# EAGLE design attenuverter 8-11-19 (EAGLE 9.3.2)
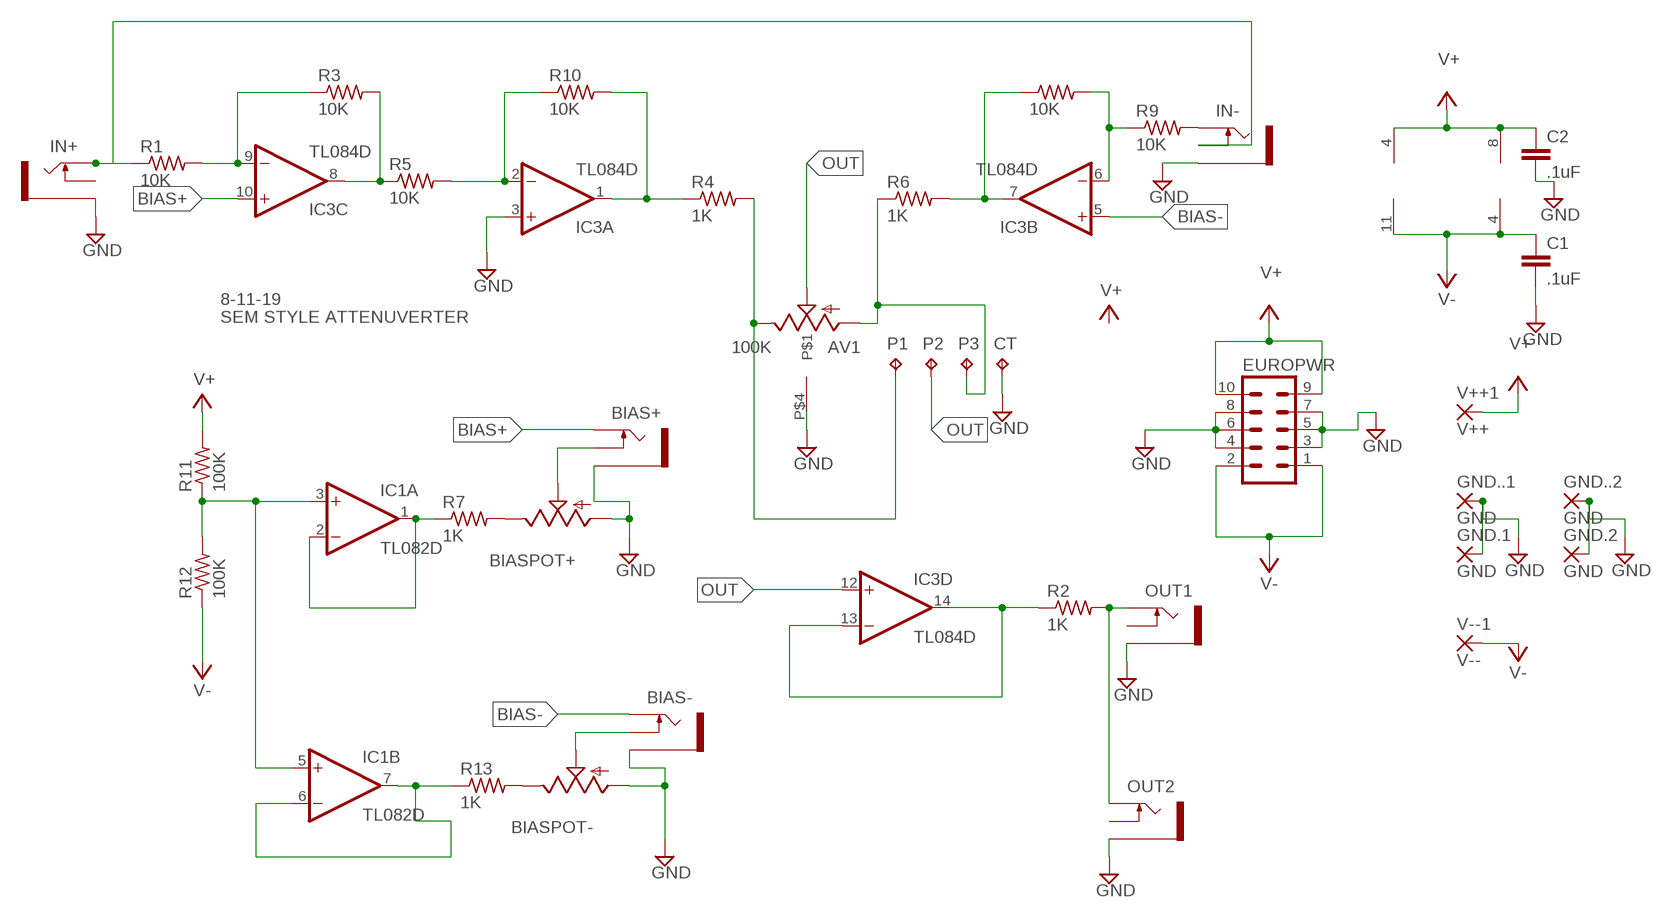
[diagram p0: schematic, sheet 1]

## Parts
AV1  100K  ALPSRK11K114  [ALPSCENTERTAP]
BIAS+  THONKICONNOLD  [THONKICONN]
BIAS-  THONKICONNOLD  [THONKICONN]
BIASPOT+  9MM_SNAP-IN_POT_  [9MM_SNAP-IN_POT]
BIASPOT-  9MM_SNAP-IN_POT_  [9MM_SNAP-IN_POT]
C1  .1uF  C5/3.5  [C5B3.5]
C2  .1uF  C5/3.5  [C5B3.5]
CT  TPPAD1-13  [P1-13]
EUROPWR  EURO_POWER_HEADERREGULAR  [EURO_POWER_HEADER]
GND.1  GND  1,6/0,8  [1,6/0,8]
GND.2  GND  1,6/0,8  [1,6/0,8]
GND..1  GND  1,6/0,8  [1,6/0,8]
GND..2  GND  1,6/0,8  [1,6/0,8]
IC1  TL082D  [SO08]
IC3  TL084D  [SO14]
IN+  THONKICONNOLD  [THONKICONN]
IN-  THONKICONNOLD  [THONKICONN]
OUT1  THONKICONNOLD  [THONKICONN]
OUT2  THONKICONNOLD  [THONKICONN]
P1  TPPAD1-13  [P1-13]
P2  TPPAD1-13  [P1-13]
P3  TPPAD1-13  [P1-13]
R1  10K  R-US_0204/7  [0204/7]
R2  1K  R-US_0204/7  [0204/7]
R3  10K  R-US_0204/7  [0204/7]
R4  1K  R-US_0204/7  [0204/7]
R5  10K  R-US_0204/7  [0204/7]
R6  1K  R-US_0204/7  [0204/7]
R7  1K  R-US_0204/7  [0204/7]
R8  10K  R-US_0204/7  [0204/7]
R9  10K  R-US_0204/7  [0204/7]
R10  10K  R-US_0204/7  [0204/7]
R11  100K  R-US_0204/7  [0204/7]
R12  100K  R-US_0204/7  [0204/7]
R13  1K  R-US_0204/7  [0204/7]
V++1  V++  1,6/0,8  [1,6/0,8]
V--1  V--  1,6/0,8  [1,6/0,8]

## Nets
BIAS+: BIAS+.P$3_TIP(TIP) IC3.10(C:+IN)
BIAS-: BIAS-.P$3_TIP(TIP) IC3.5(B:+IN)
GND: AV1.P$4 BIAS+.P$1_SLEEVE(SLEEVE) BIAS-.P$1_SLEEVE(SLEEVE) BIASPOT+.1(A) BIASPOT-.1(A) C1.2 C2.2 CT.TP EUROPWR.3 EUROPWR.4 EUROPWR.5 EUROPWR.6 EUROPWR.7 EUROPWR.8 GND.1.1(P) GND.2.1(P) GND..1.1(P) GND..2.1(P) IC3.3(A:+IN) IN+.P$1_SLEEVE(SLEEVE) IN-.P$1_SLEEVE(SLEEVE) OUT1.P$1_SLEEVE(SLEEVE) OUT2.P$1_SLEEVE(SLEEVE)
N$1: IC3.6(B:-IN) R8.2 R9.1
N$2: IC1.3(A:+IN) IC1.5(B:+IN) R11.1 R12.2
N$3: IC3.7(B:OUT) R6.2 R8.1
N$4: IC1.1(A:OUT) IC1.2(A:-IN) R7.1
N$5: AV1.P$1(HIGH) P1.TP R4.2
N$6: IC1.6(B:-IN) IC1.7(B:OUT) R13.1
N$7: BIASPOT-.3(E) R13.2
N$8: IN-.P$3_TIP(TIP) R9.2
N$9: BIAS+.P$2_SWITCH(SWITCH) BIASPOT+.2(S)
N$10: BIAS-.P$2_SWITCH(SWITCH) BIASPOT-.2(S)
N$11: IC3.9(C:-IN) R1.2 R3.1
N$12: IC3.13(D:-IN) IC3.14(D:OUT) R2.1
N$13: AV1.P$3(LOW) P3.TP R6.1
N$14: BIASPOT+.3(E) R7.2
N$16: IC3.8(C:OUT) R3.2 R5.1
N$17: IC3.2(A:-IN) R5.2 R10.1
N$18: IC3.1(A:OUT) R4.1 R10.2
N$19: IN+.P$3_TIP(TIP) IN-.P$2_SWITCH(SWITCH) R1.1
N$20: OUT1.P$3_TIP(TIP) OUT2.P$3_TIP(TIP) R2.2
OUT: AV1.P$2(WIPER) IC3.12(D:+IN) P2.TP
V+: C2.1 EUROPWR.9 EUROPWR.10 IC1.8(P:V+) IC3.4(P:V+) R11.2 V++1.1(P)
V-: C1.1 EUROPWR.1 EUROPWR.2 IC1.4(P:V-) IC3.11(P:V-) R12.1 V--1.1(P)
Unconnected: IN+.P$2_SWITCH(SWITCH) OUT1.P$2_SWITCH(SWITCH) OUT2.P$2_SWITCH(SWITCH)

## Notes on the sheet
- 8-11-19
- SEM STYLE ATTENUVERTER

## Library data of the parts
AV1 = MusicThingModular-CL:ALPSRK11K114: ALPS Pot with center tap ground
BIAS+ BIAS- IN+ IN- OUT1 OUT2 = MusicThingModular:THONKICONN: 3.5mm socket for Eurorack modular synths
BIASPOT+ BIASPOT- = MusicThingModular:9MM_SNAP-IN_POT: 9mm vertical snap-in pot, Alpha / Panasonic style
C1 C2 = capacitor-wima:C: CAPACITOR
CT P1-P3 = testpad-CL:TP: Test pad NO NAME
EUROPWR = MusicThingModular:EURO_POWER_HEADER: Power Header 10 pin power header for Eurorack Power Supplies Variants with fatter pads for easier soldering, and the LOCK variant which has 5mil offset pins to hold the component in place before soldering
GND.1 GND.2 GND..1 GND..2 V++1 V--1 = wirepad-NONAMES:1,6/0,8: THROUGH-HOLE PAD
IC1 = linear:TL082: OP AMP Data sheet; DATA_SHEET: <a href="http://www.ti.com/lit/ds/symlink/tl084a.pdf"> Data sheet </a>
IC3 = linear:TL084: OP AMP
R1-R13 = rcl:R-US_: RESISTOR, American symbol

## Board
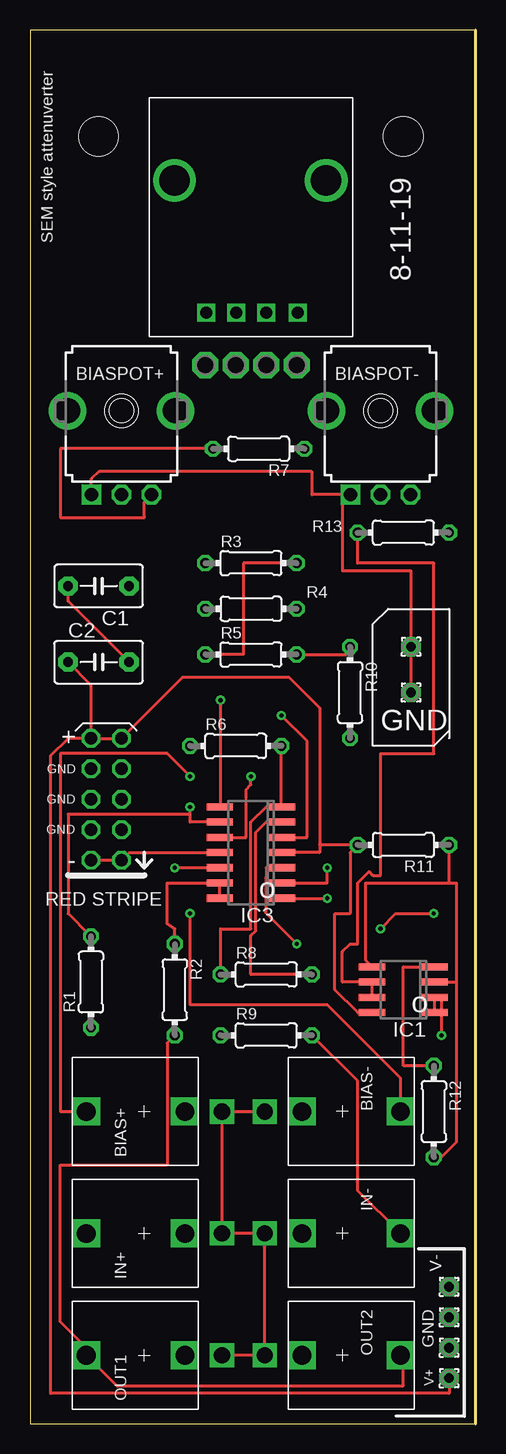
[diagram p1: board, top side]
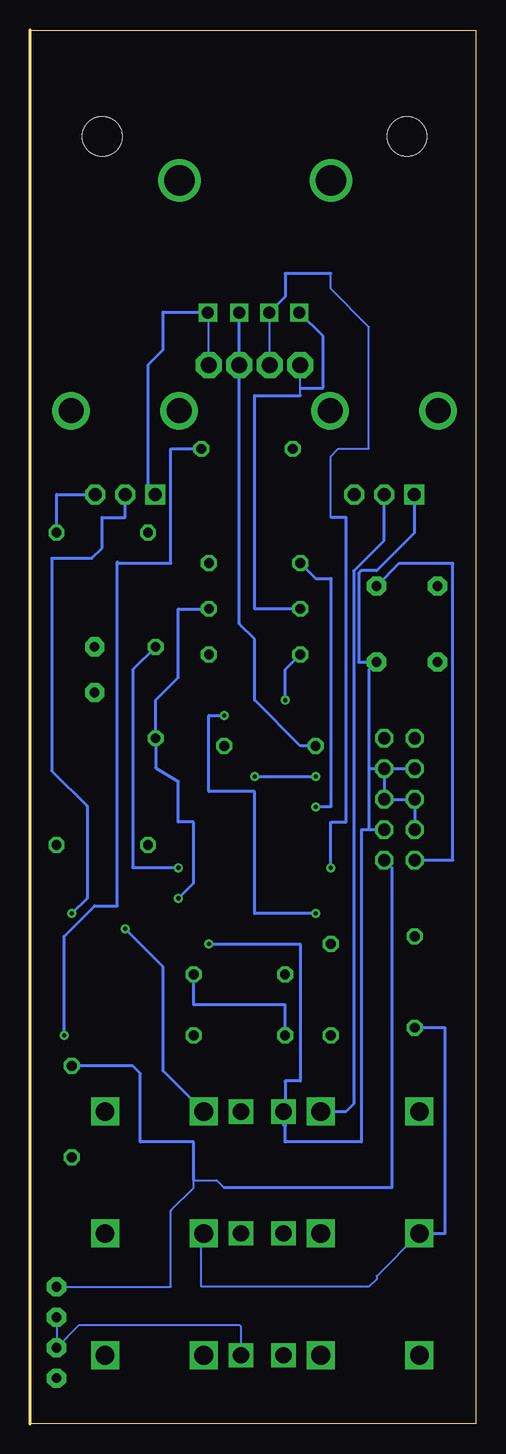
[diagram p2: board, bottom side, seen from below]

Size 37.14 x 116.19 mm. Coordinates in mm from the lower left corner, seen from the top.
Outline: 0,0 37.14,0 37.14,116.19 0,116.19 0,0
Copper layers (1*16): Top 0.035mm / dielectric 1.5mm / Bottom 0.035mm
Design rules "default": minimum track width 6mil, minimum drill 0.35mm, track to track 6mil, track to pad 6mil, pad to pad 6mil, via to via 6mil, smd to smd 6mil, copper to edge 40mil, drill to drill 6mil, minimum pad ring 10mil, minimum via ring 8mil, stop-mask expansion 4mil, vias tented up to drill 0mil, thermal gap 10mil
Holes 3.3 mm at 5.71,107.31 31.11,107.31

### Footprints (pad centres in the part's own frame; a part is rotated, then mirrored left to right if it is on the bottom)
ALPSCENTERTAP = drill 1 square: P$1 10.238,3.746; P$2 12.738,3.746; P$3 15.238,3.746; P$4 17.857,3.746 | drill 2.54: P$5 7.603,14.746; P$6 20.238,14.746
THONKICONN = drill 1.35 square: P$1_SLEEVE 0,-6.48 | drill 1.55 square: P$2_SWITCH 0,-3.38; P$3_TIP 0,4.84
9MM_SNAP-IN_POT = drill 1.1 square: 1 -2.5,-7 | drill 1.1 octagon: 2 0,-7; 3 2.5,-7 | drill 2.1 pad 2.794: CHASSIS1 -4.5,0; CHASSIS2 4.5,0
C5B3.5 = drill 0.813 pad 1.6 octagon: 1 -2.54,0; 2 2.54,0
P1-13 = drill 1.321 pad 2.159 octagon: TP 0,0
EURO_POWER_HEADER = drill 1.016 octagon: 1 -5.08,-1.27; 2 -5.08,1.27; 3 -2.54,-1.27; 4 -2.54,1.27; 5 0,-1.27; 6 0,1.27; 7 2.54,-1.27; 8 2.54,1.27; 9 5.08,-1.27; 10 5.08,1.27
1,6/0,8 = drill 0.813 pad 1.6 octagon: 1 0,0
SO08 = smd 0.6 x 2.2: 1 -1.905,-2.6; 2 -0.635,-2.6; 3 0.635,-2.6; 4 1.905,-2.6; 5 1.905,2.6; 6 0.635,2.6; 7 -0.635,2.6; 8 -1.905,2.6
SO14 = smd 0.6 x 2.2: 1 -3.81,-2.6; 2 -2.54,-2.6; 3 -1.27,-2.6; 4 0,-2.6; 5 1.27,-2.6; 6 2.54,-2.6; 7 3.81,-2.6; 8 3.81,2.6; 9 2.54,2.6; 10 1.27,2.6; 11 0,2.6; 12 -1.27,2.6; 13 -2.54,2.6; 14 -3.81,2.6
0204/7 = drill 0.813 octagon: 1 -3.81,0; 2 3.81,0

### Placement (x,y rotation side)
AV1  4.45,88.9 0 top
BIAS+  9.53,26.04 90 top
BIAS-  26.04,26.04 270 top
BIASPOT+  7.62,84.45 0 top
BIASPOT-  29.21,84.45 0 top
C1  5.71,69.85 180 top
C2  5.71,63.5 0 top
CT  22.23,88.27 0 top
EUROPWR  6.35,52.07 90 top
GND.1  34.92,8.89 90 top
GND.2  31.75,64.77 0 top
GND..1  34.92,6.35 90 top
GND..2  31.75,60.96 0 top
IC1  31.11,36.19 90 top
IC3  18.41,47.62 90 top
IN+  9.53,15.88 90 top
IN-  26.04,15.88 270 top
OUT1  9.53,5.71 90 top
OUT2  26.04,5.71 270 top
P1  14.61,88.27 0 top
P2  17.14,88.27 0 top
P3  19.68,88.27 0 top
R1  5.08,36.83 90 top
R2  12.07,36.19 270 top
R3  18.41,71.75 0 top
R4  18.41,67.94 180 top
R5  18.41,64.13 0 top
R6  17.14,56.52 0 top
R7  19.05,81.28 180 top
R8  19.68,37.47 0 top
R9  19.68,32.39 0 top
R10  26.67,60.96 270 top
R11  31.11,48.26 180 top
R12  33.66,26.04 270 top
R13  31.11,74.3 0 top
V++1  34.92,3.81 90 top
V--1  34.92,11.43 90 top

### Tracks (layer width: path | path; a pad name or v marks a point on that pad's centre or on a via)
BIAS+  (via drill 0.35)
  Top 0.254: BIAS+.P$3_TIP 2.54,26.04 2.54,55.88 11.43,55.88 v13.34,53.97 | IC3.10 18.01,48.89 18.01,52.87 18.41,53.28 v18.41,53.97
  Bottom 0.254: v18.41,53.97 v13.34,53.97
BIAS-  (via drill 0.35)
  Top 0.254: BIAS-.P$3_TIP 30.88,28.82 24.77,34.92 13.34,34.92 v13.34,42.55 | IC3.5 23.09,48.89 23.09,56.92 v20.96,59.05
  Bottom 0.254: v13.34,42.55 18.41,42.55 18.41,52.7 22.23,52.7 22.23,59.05 v20.96,59.05
GND  (via drill 0.35)
  Top 0.254: OUT1.P$1_SLEEVE OUT2.P$1_SLEEVE IN-.P$1_SLEEVE IN+.P$1_SLEEVE BIAS+.P$1_SLEEVE BIAS-.P$1_SLEEVE | IC3.3 19.68,46.36 19.68,45.55 19.64,45.5 19.64,42.59 v22.23,40 | GND..2.1 GND.2.1 31.75,71.12 26.04,71.12 26.04,77.47 26.69,77.47 BIASPOT-.1 23.5,77.45 23.5,79.38 5.71,79.38 5.12,78.78 BIASPOT+.1 | C2.2 3.18,68.58 C1.2
  Bottom 0.152: GND.1.1 GND..1.1 33.02,8.26 19.68,8.26 19.55,8.12 OUT2.P$1_SLEEVE | CT.TP 22.23,92.57 AV1.P$4
  Bottom 0.254: BIASPOT-.1 27.31,78.05 27.31,88.27 26.04,89.53 26.04,92.71 25.97,92.65 AV1.P$4 | EUROPWR.8 EUROPWR.7 | EUROPWR.7 EUROPWR.5 EUROPWR.6 EUROPWR.4 | EUROPWR.7 8.89,54.61 | 8.89,54.61 8.89,49.53 | 8.89,49.53 9.53,49.53 9.53,23.5 15.88,23.5 15.88,24.77 | 8.89,49.53 EUROPWR.3 | 8.89,54.61 8.89,62.86 C2.2 9.75,63.5 9.75,70.89 9.53,71.12 8.26,71.12 5.12,74.25 BIASPOT+.1 | v22.23,40 14.61,40 14.61,28.57 15.88,28.57 15.88,24.77 | 15.88,24.77 16,24.89 BIAS+.P$1_SLEEVE
N$1
  Top 0.254: R8.2 18.41,37.47 18.41,40.7 18.82,41.11 18.82,49.3 19.68,50.17 IC3.6
  Bottom 0.254: R9.1 15.88,34.92 23.5,34.92 R8.2
N$2
  Top 0.254: IC1.3 35.56,36.83 | 35.56,36.83 35.56,37.47 35.56,45.08 34.92,45.08 | 34.92,45.08 R11.1 | IC1.5 27.94,38.67 27.94,45.08 34.92,45.08 | R12.2 34.29,22.23 35.56,23.5 35.56,36.83
N$3
  Top 0.254: IC3.7 20.98,51.47 | 20.98,51.47 20.96,51.5 R6.2 | R8.1 15.88,41.28 18.41,41.28 18.41,50.17 19.71,51.47 20.98,51.47
N$4  (via drill 0.35)
  Top 0.254: IC1.1 IC1.2 34.29,35.56 v34.29,32.39
  Bottom 0.254: R7.1 25.4,81.28 25.4,71.75 29.75,71.75 29.85,71.85 29.85,43.18 31.75,43.18 34.29,40.64 34.29,38.73 34.29,38.1 v34.29,32.39
N$5
  Bottom 0.152: 14.61,85.72 14.61,86.36 P1.TP
  Bottom 0.254: R4.2 18.41,67.94 18.41,85.72 14.61,85.72 | 14.61,86.36 12.7,86.36 12.7,90.66 AV1.P$1
N$6
  Top 0.254: IC1.7 IC1.6 26.04,36.83 26.04,39.37 26.67,40 27.31,40 27.31,45.08 28.26,46.04 28.57,45.72 29.21,45.72 29.21,55.88 33.66,55.88 33.66,71.75 27.31,71.75 R13.1
N$7
  Bottom 0.254: R13.2 34.92,77.47 31.72,77.47 BIASPOT-.3
N$8
  Top 0.254: IN-.P$3_TIP 27.31,19.45 27.31,28.57 R9.2
N$9
  Bottom 0.254: BIAS+.P$2_SWITCH 10.8,26.04 10.16,26.67 10.16,71.1 7.62,73.64 BIASPOT+.2
N$10  (via drill 0.35)
  Top 0.254: v29.21,41.28 30.48,42.55 v33.66,42.55
  Bottom 0.254: BIASPOT-.2 29.21,75.56 31.11,75.56 31.11,73.02 31.98,72.16 35.33,72.16 35.33,54.44 32.39,51.5 32.39,43.81 v33.66,42.55 | BIAS-.P$2_SWITCH 26.04,29.42 26.04,38.1 v29.21,41.28
N$11  (via drill 0.35)
  Top 0.254: IC3.9 13.34,50.17 13.34,50.8 | 13.34,50.8 3.18,50.8 3.18,42.55 R1.2 | 13.34,50.8 v13.34,51.44
  Bottom 0.254: v13.34,51.44 12.07,51.44 12.07,70.48 13.34,70.48 R3.1
N$12
  Top 0.254: R2.1 12.07,41.28 11.43,41.7 11.43,45.08 IC3.13 IC3.14
N$13
  Bottom 0.152: P3.TP AV1.P$3
  Bottom 0.254: R6.1 14.61,56.52 18.41,60.33 18.41,65.41 19.68,66.67 AV1.P$3
N$14
  Top 0.254: R7.2 2.54,81.28 2.54,75.56 9.53,75.56 9.53,76.86 BIASPOT+.3
N$16  (via drill 0.35)
  Top 0.254: R3.2 17.78,71.75 17.78,64.13 R5.1 | IC3.8 15.88,51.5 v15.88,60.33
  Bottom 0.254: v15.88,60.33 15.88,62.86 R5.1
N$17  (via drill 0.35)
  Top 0.254: R5.2 26.35,64.13 R10.1 | IC3.2 24.77,45.08 v24.77,46.36
  Bottom 0.254: v24.77,46.36 28.57,46.36 28.57,62.86 R10.1
N$18  (via drill 0.35)
  Top 0.254: IC3.1 v24.77,43.81
  Bottom 0.254: v24.77,43.81 23.5,45.08 23.5,50.17 24.77,50.17 24.77,53.54 26.67,54.69 R10.2 26.67,60.33 24.77,62.23 24.77,67.94 R4.1
N$19
  Bottom 0.152: IN+.P$3_TIP 8.26,12.3 8.26,12.07 8.89,11.43 22.86,11.43 22.86,15.67 IN-.P$2_SWITCH
  Bottom 0.254: IN+.P$3_TIP 2.54,15.88 2.54,33.02 R1.1
N$20
  Top 0.254: R2.2 11.43,31.75 11.43,21.59 2.54,21.59 2.54,8.5 4.69,6.35 OUT1.P$3_TIP 7.22,3.18 31.11,3.18 31.11,5.47 OUT2.P$3_TIP
OUT  (via drill 0.35)
  Top 0.254: IC3.12 v12.07,46.36
  Bottom 0.152: AV1.P$2 17.18,88.3 P2.TP | 12.07,75.56 12.07,80.64 11.43,81.28 8.89,81.28 8.89,91.44 12.07,94.61 12.07,95.88
  Bottom 0.254: 12.07,95.88 15.88,95.88 15.88,93.95 AV1.P$2 | 12.07,75.56 10.8,75.56 10.8,50.17 12.07,50.17 v12.07,46.36
V+
  Top 0.254: EUROPWR.10 3.18,57.15 1.73,55.7 1.73,2.54 34.92,2.54 V++1.1 | C2.1 5.08,61.59 EUROPWR.10 | EUROPWR.10 EUROPWR.9 12.7,62.23 21.59,62.23 24.13,59.69 24.13,48.26 | IC1.8 27.31,34.29 25.4,36.19 25.4,42.55 26.67,42.55 26.67,47.62 R11.2 24.13,48.26 | IC3.4 24.13,47.62 24.13,48.26
V-
  Top 0.254: EUROPWR.2 EUROPWR.1 8.26,47.62 IC3.11 | R12.1 31.11,29.85 31.11,38.1 IC1.4
  Bottom 0.152: V--1.1 25.4,11.43 25.4,17.78 23.5,19.68 23.5,20.32 21.59,20.32 20.96,19.68
  Bottom 0.254: EUROPWR.2 1.91,46.99 1.91,71.75 6.35,71.75 C1.1 | EUROPWR.1 6.98,46.36 6.98,19.68 20.96,19.68 | 23.5,20.32 23.5,23.5 27.94,23.5 27.94,29.21 28.57,29.85 R12.1

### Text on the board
tNames: SEM style attenuverter | 8-11-19 | GND | o | o | V- | GND | V+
